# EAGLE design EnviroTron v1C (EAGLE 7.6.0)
AUTHOR: w. boyett; CONTACT_ADDRESS: Licensed under CC-BY-SA; CONTACT_COMPANY: github.com/watsonboyett; CONTACT_PHONE: (Creative Commons, Attribution + Share Alike); REV: 1C
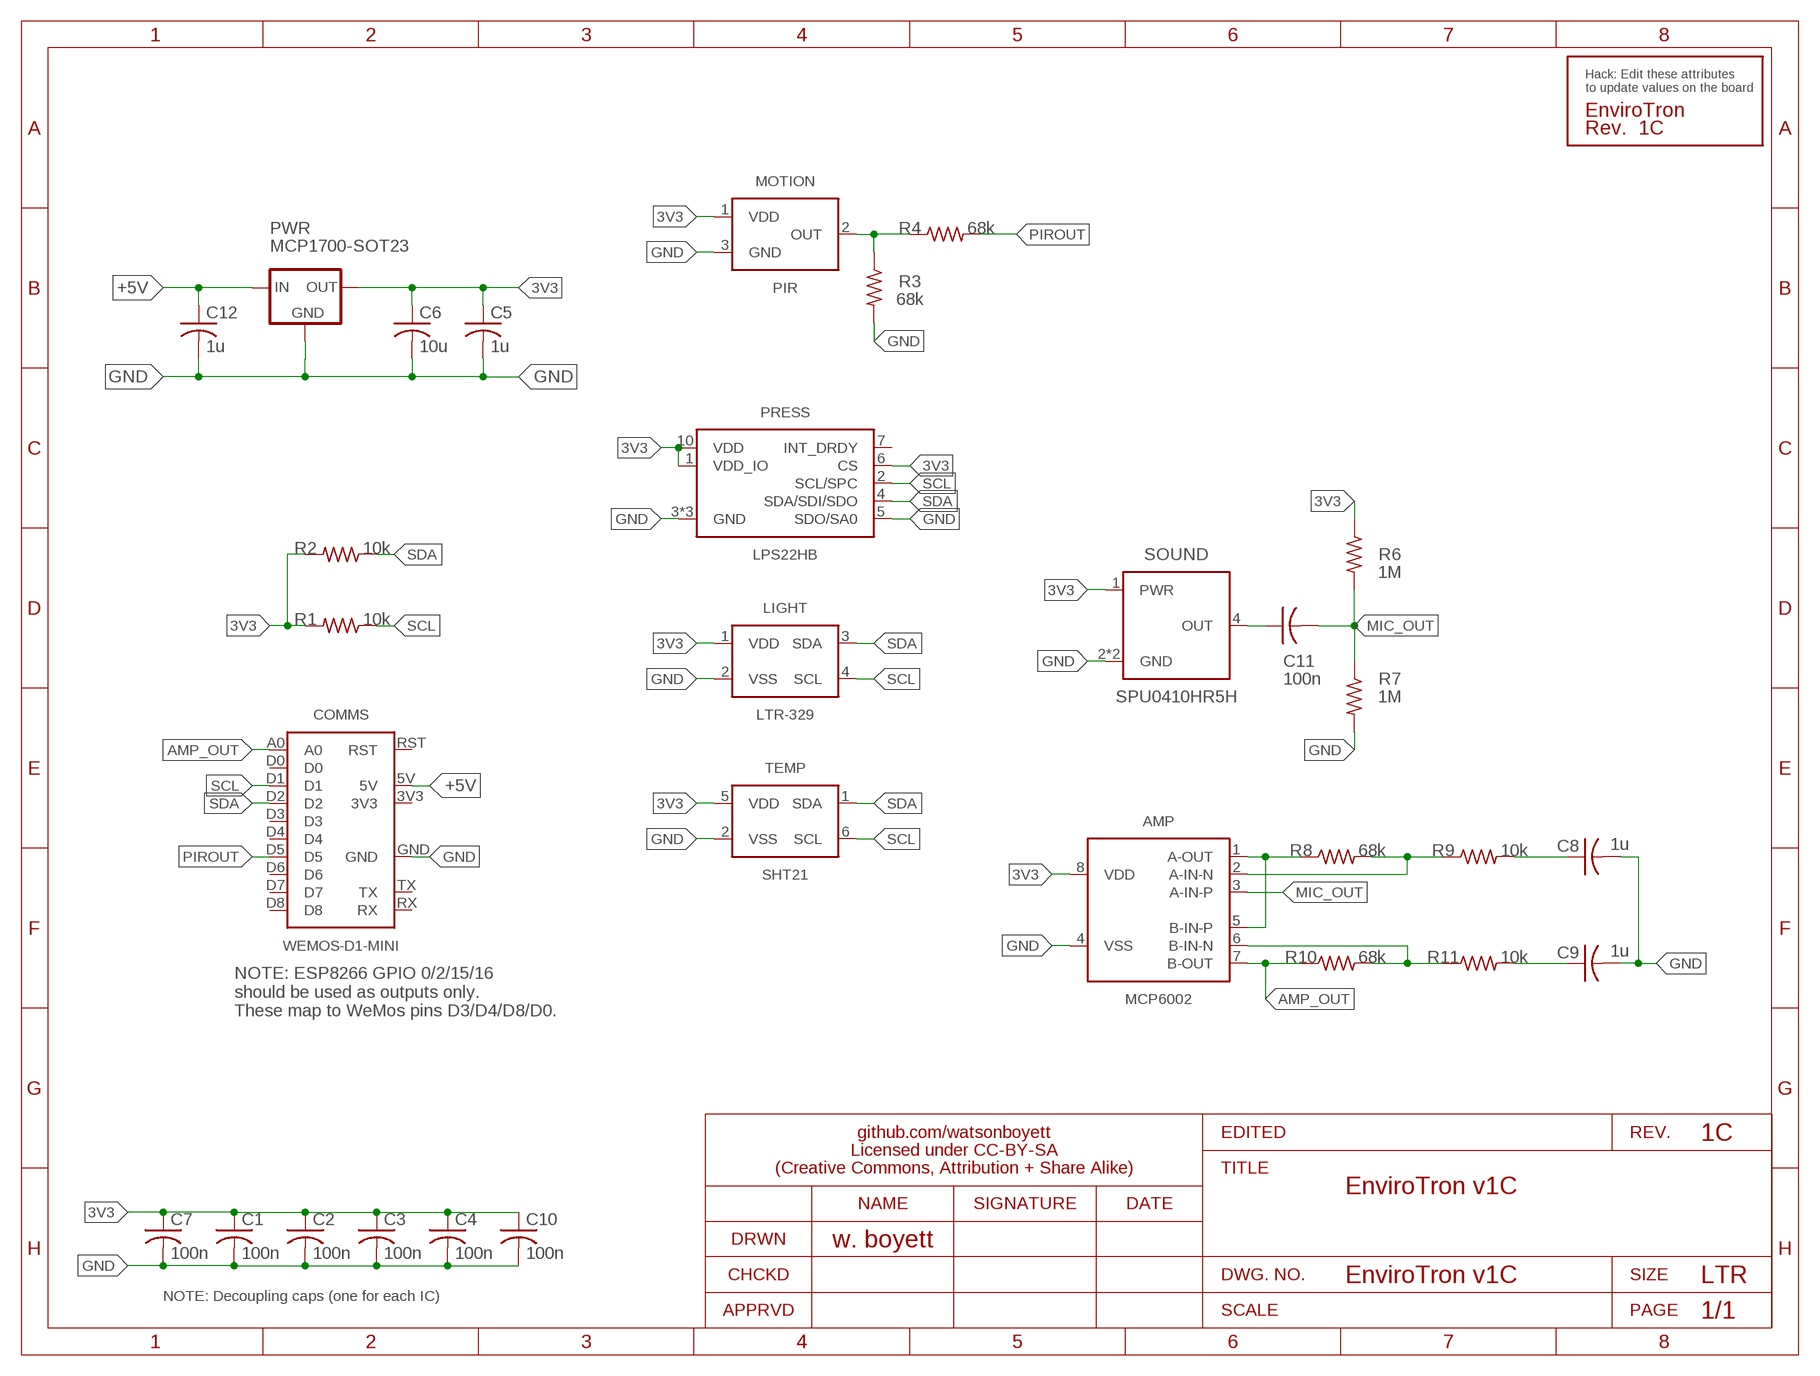
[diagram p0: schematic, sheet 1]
FRAME1 (LETTER_L): SECTION: Sensor Board

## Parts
AMP  MCP6002  [MSOP-8]
C1  100n  C-USC0603  [C0603]
C2  100n  C-USC0603  [C0603]
C3  100n  C-USC0603  [C0603]
C4  100n  C-USC0603  [C0603]
C5  1u  C-USC0603  [C0603]
C6  10u  C-USC0805  [C0805]
C7  100n  C-USC0603  [C0603]
C8  1u  C-USC0603  [C0603]
C9  1u  C-USC0603  [C0603]
C10  100n  C-USC0603  [C0603]
C11  100n  C-USC0603  [C0603]
C12  1u  C-USC0603  [C0603]
COMMS  WEMOS-D1-MINI  [WEMOS-D1-MINI]
LIGHT  LTR-329  [CHIPLED4]
MOTION  PIR  [CAN3]
PRESS  LPS22HB  [HLGA-10L]
PWR  MCP1700-SOT23  [SOT23-3]
R1  10k  R-US_R0603  [R0603]
R2  10k  R-US_R0603  [R0603]
R3  68k  R-US_R0603  [R0603]
R4  68k  R-US_R0603  [R0603]
R6  1M  R-US_R0603  [R0603]
R7  1M  R-US_R0603  [R0603]
R8  68k  R-US_R0603  [R0603]
R9  10k  R-US_R0603  [R0603]
R10  68k  R-US_R0603  [R0603]
R11  10k  R-US_R0603  [R0603]
SOUND  SPU0410HR5H  [BPAD-4]
TEMP  SHT21  [SHT2X-DFN6]
U$1  SILK_QC  [SILK_QC]

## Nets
3V3: AMP.8(VDD) C1.1 C2.1 C3.1 C4.1 C5.1 C6.1 C7.1 C10.1 LIGHT.1(VDD) MOTION.1(VDD) PRESS.1(VDD_IO) PRESS.6(CS) PRESS.10(VDD) PWR.2(OUT) R1.2 R2.2 R6.1 SOUND.1(PWR) TEMP.5(VDD)
+5V: C12.1 COMMS.5V PWR.3(IN)
AMP_OUT: AMP.7(B-OUT) COMMS.A0 R10.1
GND: AMP.4(VSS) C1.2 C2.2 C3.2 C4.2 C5.2 C6.2 C7.2 C8.2 C9.2 C10.2 C12.2 COMMS.GND LIGHT.2(VSS) MOTION.3(GND) PRESS.3(GND) PRESS.5(SDO/SA0) PRESS.8(GND) PRESS.9(GND) PWR.1(GND) R3.2 R7.2 SOUND.2(GND) SOUND.3(GND) TEMP.2(VSS)
MIC_OUT: AMP.3(A-IN-P) C11.2 R6.2 R7.1
N$2: AMP.1(A-OUT) AMP.5(B-IN-P) R8.1
N$3: MOTION.2(OUT) R3.1 R4.1
N$6: AMP.2(A-IN-N) R8.2 R9.1
N$7: C8.1 R9.2
N$8: C11.1 SOUND.4(OUT)
N$9: AMP.6(B-IN-N) R10.2 R11.1
N$10: C9.1 R11.2
PIROUT: COMMS.D5 R4.2
SCL: COMMS.D1 LIGHT.4(SCL) PRESS.2(SCL/SPC) R1.1 TEMP.6(SCL)
SDA: COMMS.D2 LIGHT.3(SDA) PRESS.4(SDA/SDI/SDO) R2.1 TEMP.1(SDA)
Unconnected: COMMS.3V3 COMMS.D0 COMMS.D3 COMMS.D4 COMMS.D6 COMMS.D7 COMMS.D8 COMMS.RST COMMS.RX COMMS.TX PRESS.7(INT_DRDY)

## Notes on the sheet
- NOTE: ESP8266 GPIO 0/2/15/16 
  should be used as outputs only. 
  These map to WeMos pins D3/D4/D8/D0.
- NOTE: Decoupling caps (one for each IC)

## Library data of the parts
AMP = EnviroTron:MCP6002: IC OPAMP General Purpose Amplifier Circuit Rail-to-Rail; MFG: Microchip Technology; MPN: MCP6002T-I/MS; PN-DK: MCP6002T-I/MSCT-ND
C1-C12 = EnviroTron:C-US: CAPACITOR, American symbol
COMMS = EnviroTron:WEMOS-D1-MINI
LIGHT = EnviroTron:LTR-329: AMBIENT LIGHT PHOTO SENSOR Optical Sensor Ambient I²C; MFG: Lite-On Inc.; MPN: LTR-329ALS-01; PN-DK: 160-2160-1-ND
MOTION = EnviroTron:PIR: Sensor Motion, Pyroelectric, PIR (Passive Infrared) 197" (5m) 16.4' Polyethylene, Black Lens; MFG: Panasonic Electric Works; MPN: EKMC1601112; PN-DK: 255-3075-ND
PRESS = EnviroTron:LPS22HB: Pressure Sensor 3.77 PSI ~ 18.27 PSI (26 kPa ~ 126 kPa) Absolute 24 bit; MFG: STMicroelectronics; MPN: LPS22HBTR; PN-DK: 497-16265-1-ND
PWR = EnviroTron:MCP1700: IC Linear Voltage Regulator IC Positive Fixed Output 3.3V 250mA; MFG: Microchip Technology; MPN: MCP1700T-3302E/TT; PN-DK: MCP1700T3302ETTCT-ND
R1-R4 R6-R11 = EnviroTron:R-US_: RESISTOR, American symbol
SOUND = EnviroTron:SPU0410HR5H: MEMS MIC Analog 100Hz ~ 10kHz (Silicon) 1.5 ~ 3.6V Omnidirectional (-42dB ±3dB @ 94dB SPL); MFG: Knowles; MPN: SPU0410HR5H-PB; PN-DK: 423-1138-6-ND
TEMP = EnviroTron:SHT21: SENSOR Humidity/Temperature 3V I2C 2%; MFG: Sensirion AG; MPN: SHT21; PN-DK: 1649-1005-1-ND
U$1 = EnviroTron:SILK_QC: Model/Version Tag Silkscreen; MPN: DNP; PRODUCT: EnviroTron; REV: 1C

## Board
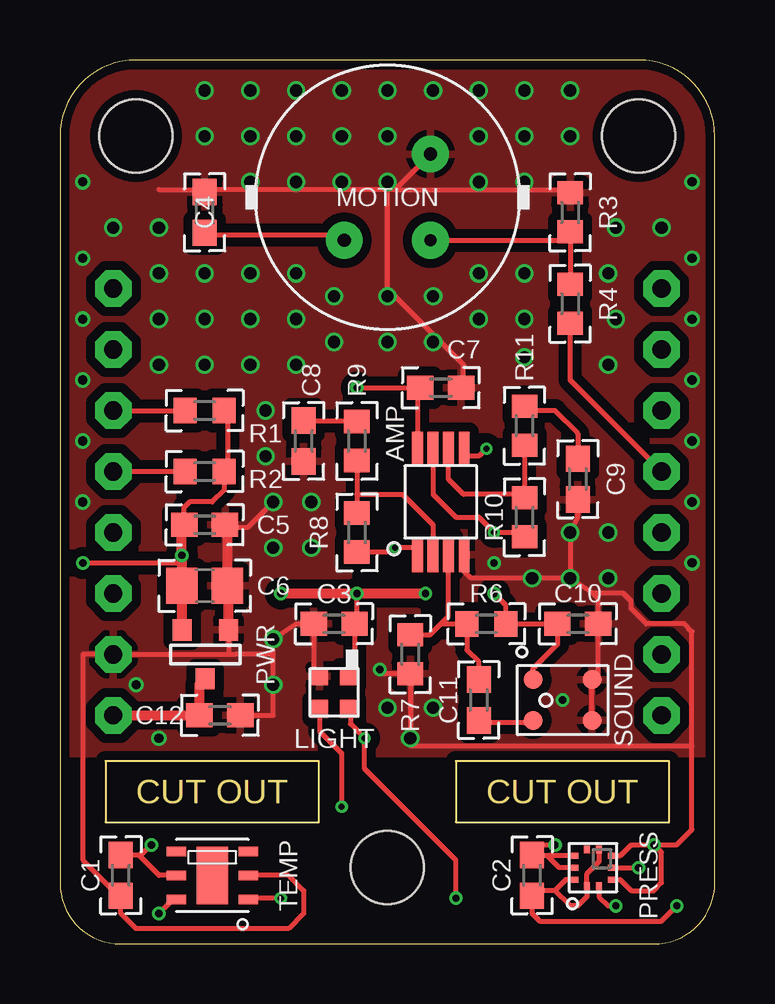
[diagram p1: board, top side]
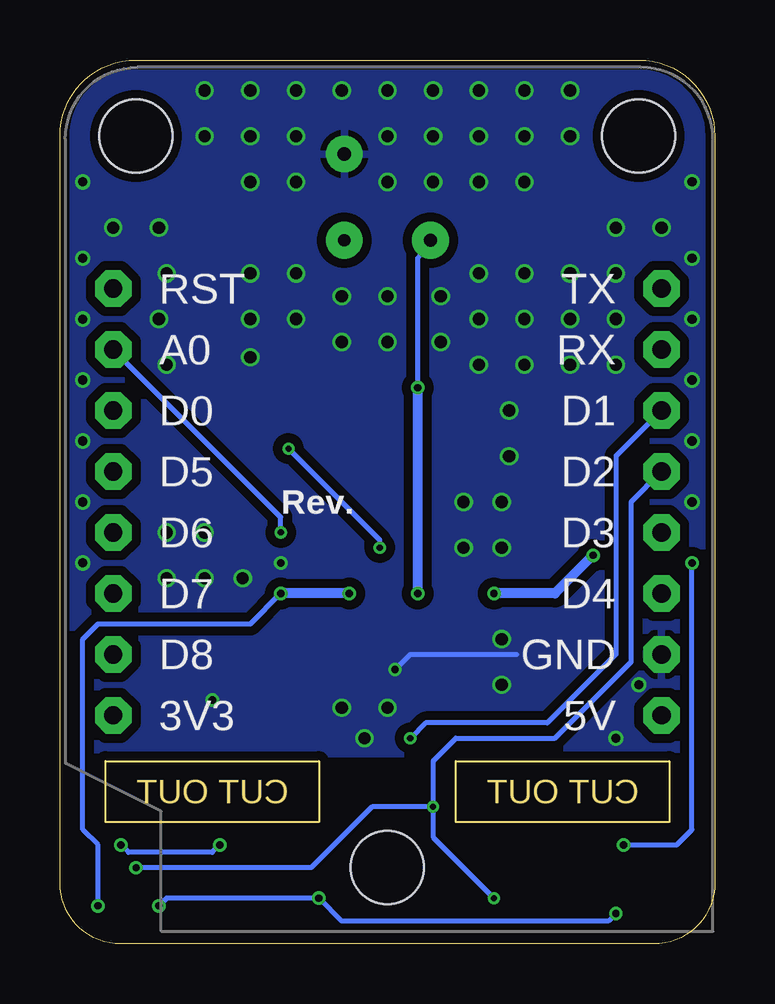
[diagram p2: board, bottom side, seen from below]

Size 27.3 x 36.83 mm. Coordinates in mm from the lower left corner, seen from the top.
Outline: 24.13,36.83 3.17,36.83 arc90 0,33.66 0,2.54 arc90 2.54,0 24.77,0 arc90 27.3,2.54 27.3,33.66 arc90 24.13,36.83
Outline: 1.91,7.62 1.91,5.08 10.79,5.08 10.79,7.62 1.91,7.62
Outline: 16.51,7.62 16.51,5.08 25.4,5.08 25.4,7.62 16.51,7.62
Copper layers (1*16): Top 0.035559375mm / dielectric 1.6mm / Bottom 0.035559375mm
Design rules "oshpark-2layer-tented *": minimum track width 8mil, minimum drill 10mil, track to track 6mil, track to pad 6mil, pad to pad 6mil, via to via 6mil, smd to smd 6mil, copper to edge 15mil, drill to drill 6mil, minimum pad ring 5mil, minimum via ring 5mil, stop-mask expansion 2.5mil, vias tented up to drill 20mil, thermal gap 10mil
Holes 3.05 mm at 3.17,33.66 24.13,33.66 13.65,3.17

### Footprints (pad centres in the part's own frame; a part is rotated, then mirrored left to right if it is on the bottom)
MSOP-8 = smd 0.45 x 1.45: 1 -0.975,-2.2; 2 -0.325,-2.2; 3 0.325,-2.2; 4 0.975,-2.2; 5 0.975,2.2; 6 0.325,2.2; 7 -0.325,2.2; 8 -0.975,2.2
C0603 = smd 1.1 x 1: 1 -0.85,0; 2 0.85,0
C0805 = smd 1.3 x 1.5: 1 -0.95,0; 2 0.95,0
WEMOS-D1-MINI = drill 0.762 pad 1.524 octagon: 3V3 -11.43,-8.89; 5V 11.43,-8.89; A0 -11.43,6.35; D0 -11.43,3.81; D1 11.43,3.81; D2 11.43,1.27; D3 11.43,-1.27; D4 11.43,-3.81; D5 -11.43,1.27; D6 -11.43,-1.27; D7 -11.43,-3.81; D8 -11.43,-6.35; GND 11.43,-6.35; RST -11.43,8.89; RX 11.43,6.35; TX 11.43,8.89
CHIPLED4 = smd 0.7 x 0.75: 1 -0.6,-0.675; 2 0.6,-0.675; 3 0.6,0.675; 4 -0.6,0.675
CAN3 = drill 0.559 pad 1.524: 1 -1.796,-1.796; 3 1.796,1.796 | drill 0.508 pad 1.524: 2 1.796,-1.796
HLGA-10L = smd 0.3 x 0.25: 1 -0.762,0.25; 2 -0.762,-0.25; 6 0.762,-0.25; 7 0.762,0.25 | smd 0.25 x 0.3: 3 -0.5,-0.762; 4 0,-0.762; 5 0.5,-0.762; 8 0.5,0.762; 9 0,0.762; 10 -0.5,0.762
SOT23-3 = smd 0.889 x 0.787: 1 1.016,-0.991; 2 1.016,0.94; 3 -1.016,-0.025
R0603 = smd 0.965 x 1.067: 1 -0.813,0; 2 0.813,0
BPAD-4 = smd 0.8 x 0.8: 1 0.85,1.23; 2 0.85,-1.23; 3 -0.85,-1.23; 4 -0.85,1.23
SHT2X-DFN6 = smd 0.4 x 0.8: 1 -1,-1.5; 2 0,-1.5; 3 1,-1.5; 4 1,1.5; 5 0,1.5; 6 -1,1.5 | smd 2.4 x 1.3: 7 0,0

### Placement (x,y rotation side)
AMP  15.88,18.41 0 top
C1  2.54,2.86 270 top
C2  19.68,2.86 90 top
C3  11.43,13.34 180 top
C4  6.03,30.48 90 top
C5  6.03,17.46 0 top
C6  6.03,14.92 0 top
C7  15.88,23.18 0 top
C8  10.16,20.95 270 top
C9  21.59,19.37 270 top
C10  21.59,13.34 0 top
C11  17.46,10.16 90 top
C12  6.67,9.53 0 top
COMMS  13.65,18.41 0 bottom
LIGHT  11.43,10.48 180 top
MOTION  13.65,31.11 0 top
PRESS  22.23,3.17 90 top
PWR  6.03,12.06 90 top
R1  6.03,22.23 0 top
R2  6.03,19.68 0 top
R3  21.27,30.48 90 top
R4  21.27,26.67 270 top
R6  17.78,13.34 180 top
R7  14.61,12.06 270 top
R8  12.38,17.14 90 top
R9  12.38,20.95 90 top
R10  19.37,17.78 90 top
R11  19.37,21.59 90 top
SOUND  20.95,10.16 90 top
TEMP  6.35,2.86 90 top
U$1  18.1,17.14 0 bottom

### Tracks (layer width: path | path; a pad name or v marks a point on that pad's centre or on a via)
3V3  (via drill 0.3)
  Top 0.203: PRESS.10 21.09,2.67 20.64,2.22 | 20.64,2.22 19.9,2.22 C2.1 19.68,1.27 20,0.95 25.08,0.95 v25.72,1.59 | 20.64,2.22 21.27,1.59 21.59,1.59 21.98,1.97 PRESS.1 21.98,2.92 22.48,3.42 PRESS.6 | TEMP.5 4.13,2.86 3.28,3.71 | 3.28,3.71 C1.1 2.54,3.49 | AMP.8 14.92,20.64 14.92,23.18 C7.1 v12.38,23.18 | C4.1 6.03,29.53 11.75,29.53 MOTION.1 | R1.2 6.99,22.23 6.99,19.68 R2.2 6.84,18.91 6.35,18.41 5.4,18.41 5.18,18.2 C5.1 | SOUND.1 19.73,11.47 20.74,12.48 C10.1 R6.1 18.59,14.11 v18.1,14.61 | LIGHT.1 12.28,11.4 C3.1 12.38,13.34 v12.38,14.61 | 3.28,3.71 3.39,3.71 v3.81,4.13 | v0.95,15.88 5.08,15.88 v5.08,16.19
  Top 0.406: v9.21,14.61 v12.38,14.61 v15.24,14.61 | C5.1 5.08,17.36 v5.08,16.19 5.08,15.88 C6.1 5.09,14.91 PWR.2
  Bottom 0.203: v12.38,23.18 12.38,28.57 MOTION.1 | v3.81,4.13 1.59,4.13 0.95,4.76 v0.95,15.88 | v25.72,1.59 25.72,4.13 26.35,4.76 26.35,12.7 25.72,13.34 23.81,13.34 21.27,13.34 19.37,13.34 v18.1,14.61
  Bottom 0.406: v12.38,14.61 v12.38,23.18 | v5.08,16.19 6.67,14.61 v9.21,14.61 | v15.24,14.61 v18.1,14.61
+5V
  Top 0.406: COMMS.5V C12.1 5.82,10.81 PWR.3
AMP_OUT  (via drill 0.25)
  Top 0.203: R10.1 19.68,17.14 v18.1,17.14 17.46,17.78 16.51,17.78 15.56,18.73 15.56,20.32 AMP.7
  Bottom 0.203: v18.1,17.14 18.1,17.78 COMMS.A0
GND  (via drill 0.3, 0.38, 0.51)
  Top 0.203: PRESS.8 20.32,3.67 | 20.32,3.67 19.68,3.67 C2.2 19.68,3.81 20,4.13 v20.64,4.13 | PRESS.9 20.82,3.17 20.32,3.67 | PRESS.5 23.36,3.67 23.81,4.13 v24.77,4.13 | v24.77,4.13 25.08,3.81 25.08,2.54 24.77,2.22 23.81,2.22 23.36,2.67 PRESS.3 | C9.2 21.59,17.78 v21.27,17.14 v21.27,15.24 | v21.27,15.24 20.32,15.24 17.14,15.24 16.83,15.56 AMP.4 | TEMP.2 9.53,2.86 10.16,2.22 10.16,1.27 9.53,0.64 3.17,0.64 2.54,1.27 2.54,1.91 | 13.97,31.43 21.27,31.43 R3.2 | 13.97,31.43 13.65,31.43 | 13.65,31.43 6.03,31.43 | C7.2 16.83,23.18 16.83,24.13 13.65,27.3 13.65,31.43 | 2.54,1.91 0.95,3.49 0.95,12.06 COMMS.GND 6.99,12.06 | 4.13,31.43 6.03,31.43 | 6.03,31.43 C4.2 | MOTION.3 13.97,31.43 | SOUND.3 SOUND.2 22.44,11.01 C10.2 22.44,14.39 22.23,14.61 | 6.99,12.06 7.3,12.06 8.89,12.06 | LIGHT.2 10.58,11.4 C3.2 9.84,13.34 v8.89,12.7 8.89,12.06 | 2.54,1.91 C1.2 | v24.77,4.13 25.72,4.13 26.35,4.76 26.35,8.26 | 26.35,8.26 26.35,13.02 26.04,13.34 24.45,13.34 23.81,13.97 23.81,14.29 23.5,14.61 22.23,14.61 | v13.34,11.43 13.51,11.25 R7.2 14.61,9.84 14.61,8.26 26.35,8.26 | 22.23,14.61 v21.27,15.24 | 6.98,17.36 7.84,17.36 8.26,17.78 8.68,18.2 | C12.2 8.89,9.53 8.89,12.06 | PWR.1 7.02,12.1 6.99,12.06
  Top 0.406: PWR.1 7.02,14.88 C6.2 6.98,17.36 C5.2
  Bottom 0.203: v20.64,4.13 20.95,3.81 24.45,3.81 v24.77,4.13 | v13.34,11.43 12.7,12.06 8.26,12.06
  other vias: 4.13,24.13 4.13,27.94 4.13,26.04 6.03,35.56 21.27,33.66 17.46,26.04 6.03,26.04 6.03,27.94 6.03,24.13 7.94,26.04 7.94,27.94 7.94,24.13 9.84,24.13 9.84,26.04 19.37,26.04 19.37,24.45 19.37,27.94 6.03,33.66 7.94,33.66 7.94,35.56 9.84,35.56 19.37,33.66 19.37,35.56 17.46,35.56 21.27,35.56 23.18,26.04 22.86,24.13 22.86,27.94 23.18,29.84 25.08,29.84 4.13,29.84 2.22,29.84 15.56,26.99 13.65,25.08 8.89,10.79 8.57,22.23 8.57,20.32 18.1,15.88 19.68,15.24 22.86,17.14 14.61,8.57 13.65,9.84 15.56,9.84 8.89,18.41 9.84,33.66 11.75,35.56 13.65,35.56 15.56,35.56 11.75,33.66 13.65,33.66 17.46,33.66 7.94,31.75 9.84,31.75 11.75,31.75 13.65,31.75 17.46,31.75 19.37,31.75 17.46,27.94 13.65,26.99 15.56,25.08 20.95,10.16 10.48,18.41 8.89,16.51 10.48,16.51 11.43,26.99 11.43,25.08 9.84,27.94 22.86,15.24 0.95,18.41 0.95,20.95 0.95,23.5 0.95,26.04 0.95,28.57 26.35,28.57 26.35,26.04 26.35,23.5 26.35,20.95 26.35,18.41 26.35,15.88 0.95,31.75 26.35,31.75 4.13,8.57 3.17,10.79
  pour Top (isolate 0.381, rank 2): 0.32,0.32 0.32,36.83 26.99,36.83 26.99,0.32
  pour Bottom (isolate 0.381, rank 2): 0.32,0.32 0.32,36.83 26.99,36.83 26.99,0.32
MIC_OUT
  Top 0.203: 15.88,13.34 16.19,13.65 16.19,16.19 AMP.3 | C11.2 17.46,11.75 16.97,12.24 R6.2 15.88,13.34 | R7.1 15.42,12.88 15.88,13.34
N$1
  cutout Bottom (isolate 1.27): 0.32,7.62 26.99,7.62 26.99,0.32 0.32,0.32
  cutout Top (isolate 1.27): 0.32,7.62 26.99,7.62 26.99,0.32 0.32,0.32
N$2  (via drill 0.25)
  Top 0.203: v17.78,20.64 17.46,20.32 16.83,20.32 AMP.5 | AMP.1 14.92,16.51 14.29,16.51 v13.97,16.51 13.79,16.33 R8.1
  Bottom 0.203: v13.97,16.51 13.97,16.83 v17.78,20.64
N$3
  Top 0.203: 21.27,27.3 R4.1 R3.1 20.92,29.32 MOTION.2
N$6
  Top 0.203: R9.1 12.38,18.73 | 12.38,18.73 14.29,18.73 15.56,17.46 15.56,16.51 AMP.2 | 12.38,18.73 R8.2
N$7
  Top 0.203: C8.1 12.03,21.8 R9.2
N$8
  Top 0.203: SOUND.4 19.68,9.21 19.37,9.21 17.46,9.21 C11.1
N$9
  Top 0.203: R11.1 19.37,18.73 | 19.37,18.73 16.83,18.73 16.19,19.37 16.19,20.32 AMP.6 | 19.37,18.73 R10.2
N$10
  Top 0.203: R11.2 19.68,22.23 20.64,22.23 21.59,21.27 C9.1
PIROUT
  Top 0.203: R4.2 21.27,23.5 COMMS.D5
SCL  (via drill 0.25, 0.3)
  Top 0.203: PRESS.2 22.48,1.97 22.86,1.59 v23.18,1.59 | COMMS.D1 R1.1 | v16.51,1.91 16.51,3.49 12.7,7.3 v12.7,8.57 12.11,9.17 12.11,9.8 LIGHT.4 | TEMP.6 4.71,1.86 v4.13,1.27
  Bottom 0.203: v23.18,1.59 22.86,1.91 v16.51,1.91 15.56,0.95 4.45,0.95 v4.13,1.27 | COMMS.D1 4.13,20.32 4.13,12.06 6.99,9.21 12.06,9.21 v12.7,8.57
SDA  (via drill 0.25, 0.3)
  Top 0.203: PRESS.4 v24.13,3.17 | COMMS.D2 R2.1 | v11.75,5.71 11.75,7.94 10.83,8.86 LIGHT.3 | v9.21,1.91 7.94,1.91 TEMP.1
  Bottom 0.203: v24.13,3.17 16.83,3.17 14.29,5.71 v11.75,5.71 | v11.75,5.71 11.75,4.45 v9.21,1.91 | COMMS.D2 3.49,18.41 3.49,11.75 6.67,8.57 10.79,8.57 11.75,7.62 v11.75,5.71

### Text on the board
Dimension: CUT OUT | CUT OUT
